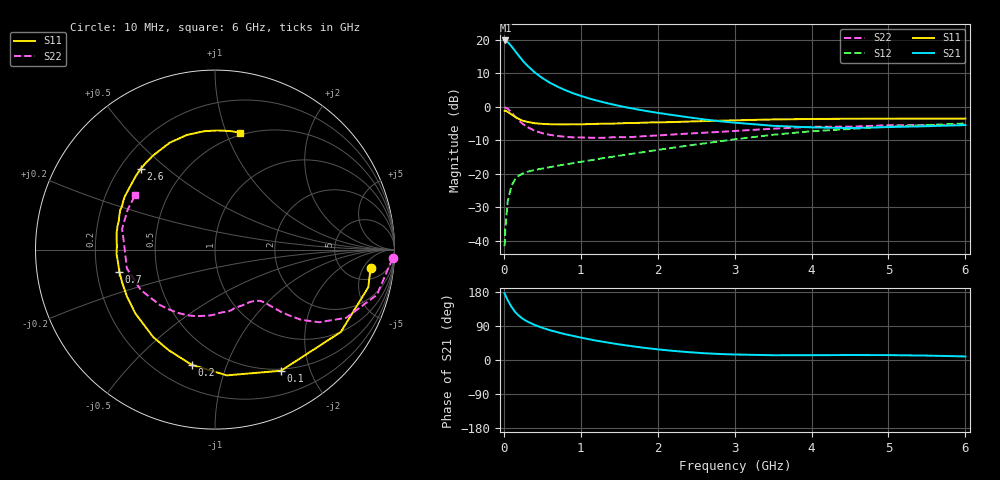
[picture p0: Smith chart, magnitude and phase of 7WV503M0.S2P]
! Infineon Technologies  Discrete & RF Semiconductors
! BFS17W
! Si NPN RF Bipolar Junction Transistor in SOT323
! VCE = 0.5 V  IC = 3 mA
! Common Emitter S-Parameters:  August  1999
# GHz  S  MA  R  50
!  f  S11  S21  S12  S22
! GHz  MAG  ANG  MAG  ANG  MAG  ANG  MAG  ANG
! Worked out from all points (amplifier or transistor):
!   36 points, 10 MHz to 6 GHz, reference 50 ohm
!   highest |S21| = 19.8 dB at 20 MHz (marker M1)
!   |S21| within 3 dB of that: start of sweep to 141.1 MHz
!   unconditionally stable (mu >= 1): 584.1 MHz to end of sweep
!   at 250 MHz: K = 0.50, MSG = 16.8 dB, |S12| = -19.9 dB
!   at 1.4 GHz: K = 1.45, MAG = 3.9 dB, |S12| = -15.0 dB
!   at 6 GHz: K = 1.15, MAG = -2.6 dB, |S12| = -5.0 dB
!   S11 on the Smith chart (normalised r, x): 10 MHz: 8, -7; 100 MHz: 0.48, -1.58; 200 MHz: 0.34, -0.76; 700 MHz: 0.30, -0.10; 2.6 GHz: 0.28, +0.41; 6 GHz: 0.48, +1.12
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0.01  0.8729 -6.8  9.76 176.1  0.0083 85.8  0.9907 -2.8
0.02  0.8795 -13.8  9.777 171.0  0.0154 84.9  0.9699 -6.4
0.05  0.8379 -33.2  9.256 157.8  0.0388 73.0  0.9367 -15.6
0.1  0.7687 -61.4  7.971 140.1  0.0664 58.2  0.8238 -27.5
0.15  0.7038 -84.6  6.713 126.0  0.0839 48.6  0.7071 -34.9
0.2  0.6551 -101.4  5.657 116.0  0.0944 43.2  0.619 -39.2
0.25  0.6171 -114.7  4.819 108.3  0.1011 39.0  0.55 -41.7
0.3  0.5966 -125.3  4.171 102.2  0.1065 37.2  0.5033 -43.4
0.4  0.5688 -141.2  3.276 92.4  0.1142 35.1  0.4391 -45.5
0.5  0.5557 -152.1  2.688 85.0  0.1195 34.7  0.4036 -46.8
0.6  0.5489 -160.4  2.276 78.6  0.1256 35.3  0.3808 -48.6
0.7  0.547 -167.1  1.991 73.1  0.1319 36.6  0.3665 -51.2
0.9  0.5494 -177.7  1.59 63.6  0.1438 38.6  0.3498 -56.9
1.1  0.5517 173.5  1.34 55.0  0.1573 40.7  0.3459 -63.8
1.3  0.5588 166.3  1.164 47.6  0.1719 42.2  0.3441 -71.6
1.6  0.572 157.4  0.976 38.2  0.1933 44.3  0.3514 -83.1
2.2  0.5916 141.9  0.751 24.1  0.2449 46.6  0.386 -106.0
2.6  0.6117 132.6  0.649 17.9  0.2833 46.4  0.4097 -120.9
3.5  0.6469 112.9  0.52 12.6  0.3822 41.3  0.4709 -151.5
4.5  0.6626 95.1  0.481 13.1  0.4659 31.0  0.505 178.0
5.5  0.666 82.6  0.513 11.6  0.5339 21.4  0.5349 155.4
6  0.6665 77.7  0.533 9.4  0.5628 16.8  0.539 145.5
